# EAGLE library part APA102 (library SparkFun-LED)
APA102 Addressable RGB LED Used in manufacturing of various products at SparkFun Packages: 5050 2020 SparkFun Products: SparkFun Lumenati Boards
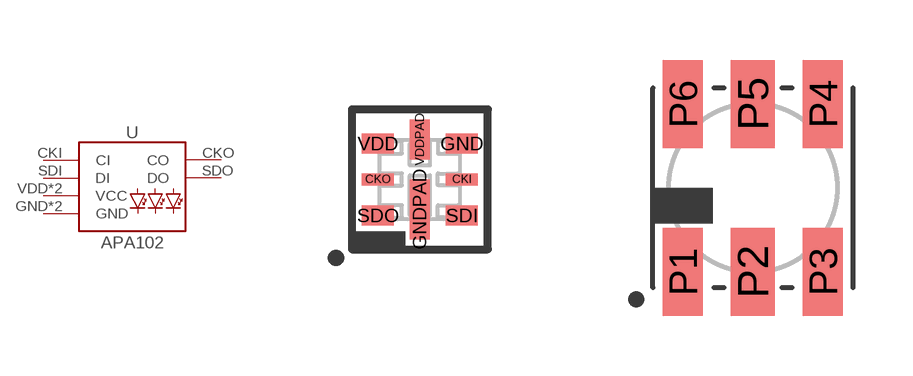
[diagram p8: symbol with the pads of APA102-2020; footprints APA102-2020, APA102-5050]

Designator prefix -

## APA1022020  [APA102-2020]
CKI  CI
CKO  CO
GND  GND
GNDPAD  GND
SDI  DI
SDO  DO
VDD  VCC
VDDPAD  VCC

## APA1025050 (PROD_ID: DIO-13739)  [APA102-5050]
P1  DI
P2  CI
P3  GND
P4  VCC
P5  CO
P6  DO

## Footprint APA102-2020 (pad centres in mm)
APA102-2020 Specifications: Pin count: 8 Size: 2.0 x 2.0 mm Datasheet referenced for footprint: APA102-2020
smd 0.8 x 0.3: CKI 1.05,0; CKO -1.05,0
smd 0.8 x 0.5: GND 1.05,0.9; SDI 1.05,-0.9; SDO -1.05,-0.9; VDD -1.05,0.9
smd 0.5 x 1.5: GNDPAD 0,-0.75
smd 0.5 x 1: VDDPAD 0,1

## Footprint APA102-5050 (pad centres in mm)
APA102C Specifications: Pin count: 6 Size: 5.0 x 5.0 mm Datasheet referenced for footprint: APA102C
smd 1 x 2.2: P1 -1.75,-2.1; P3 1.75,-2.1; P4 1.75,2.1; P6 -1.75,2.1
smd 1.1 x 2.2: P2 0,-2.1; P5 0,2.1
